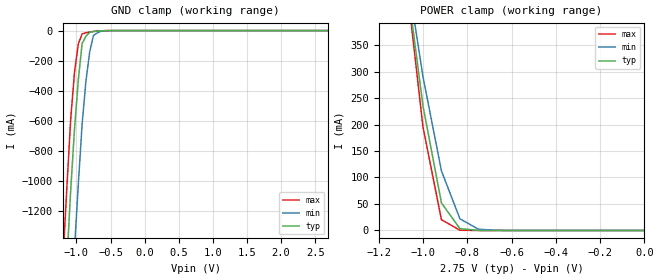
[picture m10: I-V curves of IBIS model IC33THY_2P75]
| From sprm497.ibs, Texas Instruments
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|IC33THY_3P3;
|   Model Cell IC33THY_2P75
|IC33THY_2P75
[Model]   IC33THY_2P75
Model_type   Input
Polarity   Non-Inverting
Vinl =  0.7V
Vinh =  1.7V
C_comp   0.8815254p   0.8700002p   0.8886429p
[Model Spec]
Vinl   0.7V   0.7V   0.7V
Vinh   1.7V   1.7V   1.7V
[Temperature Range]   25   125   -40
[Voltage Range]   2.75   2.475   2.89
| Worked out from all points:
|   GND clamp passes 1 mA (typ) near -0.60 V on its own axis
|   POWER clamp passes 1 mA (typ) near -0.77 V on its own axis
[POWER_clamp]
|   voltage   I(typ)   I(min)   I(max)
-2.75V    7.27A      6.178A     8.251A
-1.056V   413.2mA    440.6mA    399.5mA
-1.028V   324mA      365.4mA    297.3mA
-1V       234.9mA    290.2mA    195mA
-916.7mV  52.07mA    112.5mA    20.41mA
-833.3mV  3.49mA     22.09mA    446.6uA
-750mV    154uA      2.458mA    7.982uA
-666.7mV  6.602uA    236.3uA    142.2nA
0V        127.9pA    8.136nA    4.53pA
[GND_clamp]
|   voltage   I(typ)   I(min)   I(max)
-2.75V    -17A       -17.8A     -16.56A
-1.194V   -2.003A    -2.872A    -1.5A
-1.139V   -1.522A    -2.382A    -1.031A
-1.083V   -1.056A    -1.901A    -584.6mA
-1.028V   -651.7mA   -1.447A    -276.4mA
-972.2mV  -328.4mA   -1.021A    -88.84mA
-916.7mV  -85.95mA   -621.6mA   -21.88mA
-861.1mV  -38.15mA   -337.7mA   -15.07mA
-805.6mV  -11.53mA   -141.4mA   -9.704mA
-750mV    -6.07mA    -32.88mA   -5.786mA
-638.9mV  -1.959mA   -4.624mA   -1.428mA
2.694V    121.3pA    10.58nA    3.311pA
